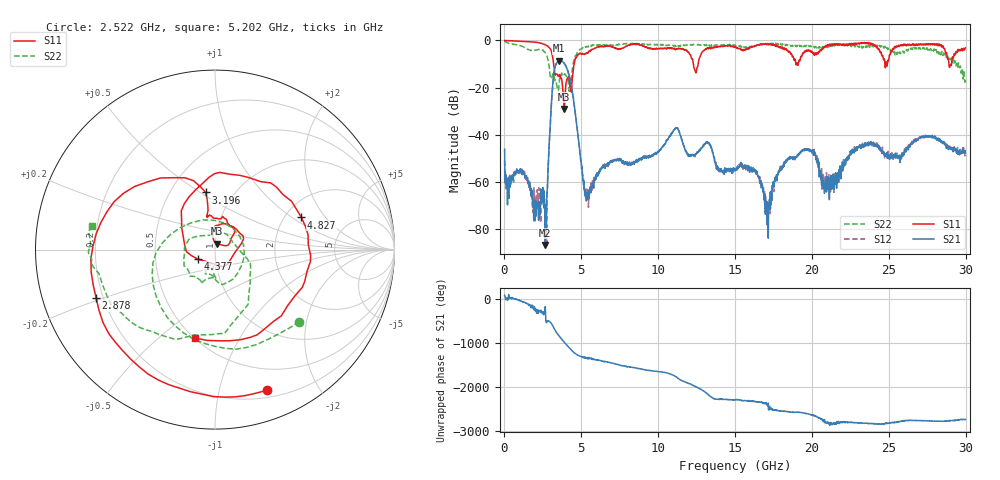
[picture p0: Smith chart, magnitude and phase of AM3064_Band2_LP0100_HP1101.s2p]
# Hz S DB R 50.0
!freq dBS11 angS11 dBS21 angS21 dBS12 angS12 dBS22 angS22
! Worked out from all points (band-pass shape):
!   1600 points, 10 MHz to 29.98 GHz, reference 50 ohm
!   highest |S21| = -8.60 dB at 3.571 GHz (marker M1); lowest = -86.6 dB at 2.653 GHz (marker M2)
!   |S21| within 3 dB of the highest: 3.278 GHz to 4.045 GHz (766.4 MHz wide, 20.9 % of centre)
!   lowest |S11| = -29.0 dB at 3.89 GHz (marker M3), VSWR 1.07, Z = 51 + j3.44 ohm
!   |S11| at or under -10 dB: 3.2 GHz to 4.536 GHz (1.336 GHz wide, 34.6 % of centre); 12.29 GHz to 12.6 GHz (311.7 MHz wide, 2.5 % of centre); 28.91 GHz to 29.08 GHz (164.6 MHz wide, 0.568 % of centre)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
!   |S22| runs from -21.6 to -0.2 dB; largest |S21 - S12| = 0.0094
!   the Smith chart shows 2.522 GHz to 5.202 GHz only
!   S11 on the Smith chart (normalised r, x): 2.522 GHz: 0.27, -1.40; 2.878 GHz: 0.17, -0.19; 3.196 GHz: 0.74, +0.53; 4.377 GHz: 0.82, -0.09; 4.827 GHz: 2.44, +1.19; 5.202 GHz: 0.50, -0.67
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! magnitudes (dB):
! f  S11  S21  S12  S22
! 10 MHz  0.0  -46.1  -50.8  -0.2
! 2.522 GHz  -1.6  -66.6  -67.5  -4.2
! 2.653 GHz  -1.9  -86.6  -72.1  -5.1
! 2.878 GHz  -2.9  -48.4  -48.4  -9.6
! 3.196 GHz  -9.8  -15.1  -15.0  -14.3
! 3.571 GHz  -14.5  -8.6  -8.6  -17.0
! 3.89 GHz  -29.0  -9.7  -9.7  -14.4
! 4.377 GHz  -19.2  -20.2  -20.1  -13.5
! 4.827 GHz  -5.8  -42.6  -42.6  -4.4
! 5.015 GHz  -5.8  -54.3  -53.0  -3.7
! 5.202 GHz  -5.9  -62.6  -63.7  -3.1
! 10 GHz  -3.5  -47.3  -47.1  -1.8
! 11.2 GHz  -3.6  -37.1  -37.0  -2.4
! 15 GHz  -2.7  -55.3  -54.7  -2.0
! 16.35 GHz  -2.3  -56.5  -55.4  -2.4
! 17.12 GHz  -1.7  -74.1  -69.9  -1.3
! 18.36 GHz  -4.2  -51.2  -50.8  -1.8
! 19.99 GHz  -4.7  -46.9  -46.9  -2.3
! 21 GHz  -1.8  -57.7  -60.8  -3.0
! 23.05 GHz  -1.1  -45.3  -45.4  -2.8
! 25 GHz  -8.2  -49.9  -48.5  -3.3
! 29.98 GHz  -3.2  -47.7  -46.4  -15.7
